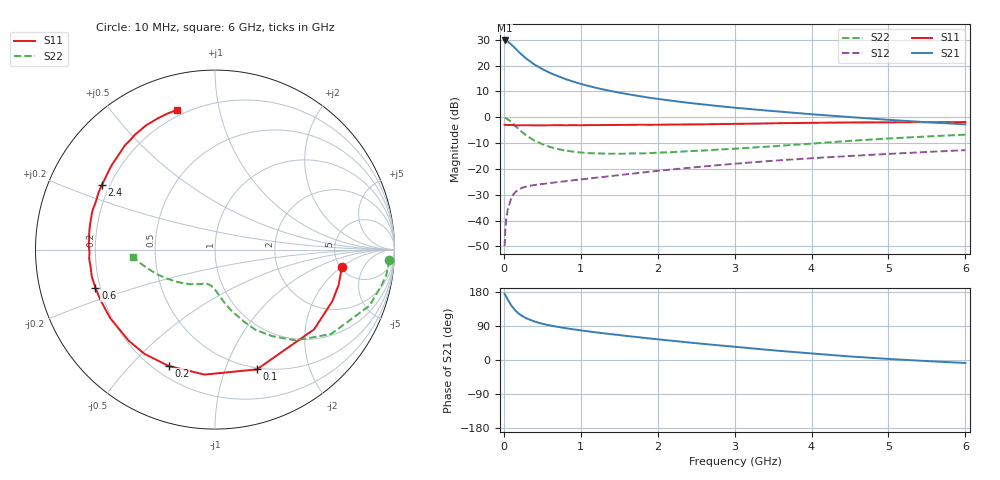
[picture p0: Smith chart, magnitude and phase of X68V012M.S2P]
! SIEMENS Small Signal Semiconductors
! BFP193W
! Si NPN RF Bipolar Junction Transistor in SOT343
! VCE = 8 V  IC = 12 mA
! Common Emitter S-Parameters:  April 1994
# GHz  S  MA  R  50
!  f  S11  S21  S12  S22
! GHz  MAG  ANG  MAG  ANG  MAG  ANG  MAG  ANG
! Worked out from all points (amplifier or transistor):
!   40 points, 10 MHz to 6 GHz, reference 50 ohm
!   highest |S21| = 29.7 dB at 10 MHz (marker M1)
!   |S21| within 3 dB of that: start of sweep to 146.5 MHz
!   unconditionally stable (mu >= 1): 1.272 GHz to 4.334 GHz
!   at 200 MHz: K = 0.24, MSG = 26.5 dB, |S12| = -27.9 dB
!   at 1.5 GHz: K = 1.06, MAG = 14.5 dB, |S12| = -22.4 dB
!   at 6 GHz: K = 0.93, MSG = 5.0 dB, |S12| = -12.7 dB
!   S11 on the Smith chart (normalised r, x): 10 MHz: 5.15, -2.03; 100 MHz: 0.48, -1.29; 200 MHz: 0.26, -0.65; 600 MHz: 0.18, -0.15; 2.4 GHz: 0.17, +0.26; 6 GHz: 0.17, +0.75
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0.01  0.7136 -7.8  30.64 174.7  0.0032 87.7  0.9724 -3.3
0.02  0.7165 -16.0  30.52 171.4  0.0069 80.9  0.9653 -8.4
0.03  0.7139 -23.8  30.23 167.5  0.0103 79.7  0.9483 -12.3
0.05  0.7088 -38.8  29.15 159.7  0.016 73.3  0.9155 -20.0
0.1  0.7071 -70.7  25.36 143.1  0.0284 58.6  0.7996 -36.0
0.15  0.6988 -94.7  21.43 130.4  0.036 49.3  0.6767 -48.4
0.2  0.6978 -111.6  18.03 121.3  0.0405 43.1  0.575 -56.8
0.25  0.7011 -124.0  15.45 114.6  0.0438 38.9  0.4985 -63.4
0.3  0.6992 -133.4  13.34 109.4  0.0459 36.8  0.4347 -67.9
0.4  0.6977 -146.7  10.46 101.5  0.0489 34.1  0.353 -74.9
0.5  0.697 -155.7  8.559 95.7  0.0511 33.5  0.3014 -79.8
0.6  0.6995 -162.3  7.211 91.2  0.0532 34.1  0.2667 -83.7
0.8  0.6997 -172.0  5.491 84.1  0.0578 35.8  0.2271 -89.1
1.1  0.7045 178.2  4.047 75.5  0.0651 39.4  0.202 -95.8
1.3  0.7066 172.7  3.434 70.4  0.0702 41.4  0.198 -99.6
1.6  0.7124 165.7  2.818 63.3  0.079 43.9  0.1978 -104.6
2.2  0.7228 153.9  2.072 50.5  0.0981 46.3  0.2117 -115.3
2.4  0.7261 150.2  1.901 46.4  0.1047 46.5  0.2204 -118.4
3.2  0.7502 136.7  1.441 31.2  0.133 45.6  0.2576 -133.2
4.5  0.7919 118.9  1.008 9.3  0.178 40.3  0.3497 -156.6
5.5  0.8021 109.8  0.801 -2.9  0.2127 35.3  0.4249 -169.9
6  0.8072 105.3  0.73 -7.9  0.231 32.9  0.4605 -175.2
